|   TEXAS INSTRUMENTS INCORPORATED
|   Standard Linear and Logic
|   IBIS Model of SN74ALVC16835
|   18-BIT Universal Bus Driver with 3-state outputs
|   56-pin DGG, DGV, or DL Package
[IBIS Ver]   2.1
[Comment char]  |_char
[File Name]   alvc16835.ibs
[File Rev]   2.0
[Date]   6/17/97
[Source]   File originated at Texas Instruments, Inc.
[Notes]   The following is an IBIS list for the ALVC16835.
|   - This file may be incomplete or may not be fully compliant
|   with the IBIS specification. It will be replaced with a
|   version that is IBIS Revision 3.2 compliant and is complete
|   and accurate.  Please email all questions and comments to
|   sllibis@ti.com
|   - All test data contained in this file are derived from
|   hspice(tm) simulations.
|   - File created by Ramzi Ammar, SLL Applications
[Disclaimer]
* Property of Texas Instruments Incorporated.  Unauthorized *
* reproduction and/or distribution is strictly prohibited. *
* This product is protected under copyright law. *
* Created 1997, (C) Copyright 1997, Texas Instruments Inc., *
* All Rights Reserved *
* UNLESS THERE IS A SIGNED, WRITTEN AGREEMENT TO THE *
* CONTRARY, TEXAS INSTRUMENTS ("TI") IS PROVIDING THE IBIS *
* MODELS "AS IS" AND WITHOUT ANY WARRANTY, EXPRESSED OR *
* IMPLIED.  TI assumes no liability for: *
* 1) the accuracy of the IBIS models provided to your *
* company; *
* 2) the proper functioning of these IBIS models in your *
* design or for any resulting applications; or *
* 3) infringement of patents, copyrights or intellectual *
* property rights resulting from your use of these *
* IBIS models. *
* TI provides IBIS Models as a service to our customers. *
* You and your company shall not distribute, sell or give *
* these models to anyone else without prior written *
* permission from TI. *
* TI reserves the right to make changes to our products or *
* to discontinue any semiconductor product or service *
* without notice, and advises our customers to obtain the *
* latest version of relevant information to verify, before *
* placing orders, that the information being relied on is *
* current. *
* Please be aware that your receipt and use of the IBIS *
* information provided shall serve as acceptance of these *
* terms and conditions.  If you do not accept these terms, *
* you should return or destroy the IBIS models and any *
* other accompanying information immediately. *
[Component]   ALVC16835_DGG
[Manufacturer]  Texas Instruments, Inc.
[Package]
|   typ   min   max
R_pkg   0.045   0.035   0.062
L_pkg   3.324nH   2.403nH   5.094nH
C_pkg   0.564pF   0.341pF   0.914pF
[Pin]   signal_name   model_name   R_pin   L_pin   C_pin
1   NC   NC   0.062   5.094nH   0.856pF
2   NC   NC   0.061   4.621nH   0.902pF
3   Y1   OUT   0.06   4.316nH   0.802pF
4   GND   GND   0.059   3.968nH   0.698pF
5   Y2   OUT   0.057   3.716nH   0.649pF
6   Y3   OUT   0.042   3.517nH   0.652pF
7   VCC   POWER   0.041   3.16nH   0.57pF
8   Y4   OUT   0.039   2.981nH   0.482pF
9   Y5   OUT   0.039   2.809nH   0.447pF
10   Y6   OUT   0.038   2.715nH   0.409pF
11   GND   GND   0.041   2.675nH   0.391pF
12   Y7   OUT   0.039   2.536nH   0.366pF
13   Y8   OUT   0.039   2.457nH   0.348pF
14   Y9   OUT   0.038   2.411nH   0.353pF
15   Y10   OUT   0.039   2.456nH   0.355pF
16   Y11   OUT   0.039   2.471nH   0.349pF
17   Y12   OUT   0.04   2.58nH   0.37pF
18   GND   GND   0.038   2.651nH   0.389pF
19   Y13   OUT   0.038   2.739nH   0.411pF
20   Y14   OUT   0.039   2.838nH   0.449pF
21   Y15   OUT   0.038   2.988nH   0.484pF
22   VCC   POWER   0.038   3.105nH   0.564pF
23   Y16   OUT   0.04   3.427nH   0.638pF
24   Y17   OUT   0.056   3.654nH   0.641pF
25   GND   GND   0.057   3.932nH   0.7pF
26   Y18   OUT   0.058   4.257nH   0.806pF
27   OE_BAR   NC   0.057   4.58nH   0.914pF
28   LE   NC   0.059   5.038nH   0.861pF
29   GND   GND   0.06   5.058nH   0.858pF
30   CLK   NC   0.056   4.543nH   0.904pF
31   A18   IN   0.057   4.24nH   0.803pF
32   GND   GND   0.057   3.929nH   0.7pF
33   A17   IN   0.056   3.616nH   0.637pF
34   A16   IN   0.037   3.368nH   0.64pF
35   VCC   POWER   0.036   3.024nH   0.563pF
36   A15   IN   0.035   2.876nH   0.474pF
37   A14   IN   0.035   2.745nH   0.444pF
38   A13   IN   0.037   2.683nH   0.405pF
39   GND   GND   0.038   2.603nH   0.382pF
40   A12   IN   0.038   2.51nH   0.362pF
41   A11   IN   0.036   2.412nH   0.341pF
42   A10   IN   0.038   2.416nH   0.349pF
43   A9   IN   0.037   2.403nH   0.349pF
44   A8   IN   0.037   2.429nH   0.341pF
45   A7   IN   0.036   2.482nH   0.358pF
46   GND   GND   0.037   2.615nH   0.381pF
47   A6   IN   0.035   2.669nH   0.402pF
48   A5   IN   0.036   2.763nH   0.442pF
49   A4   IN   0.036   2.942nH   0.478pF
50   VCC   POWER   0.035   3.053nH   0.564pF
51   A3   IN   0.036   3.409nH   0.641pF
52   A2   IN   0.058   3.698nH   0.641pF
53   GND   GND   0.059   3.975nH   0.697pF
54   A1   IN   0.061   4.327nH   0.802pF
55   NC   NC   0.061   4.624nH   0.905pF
56   GND   GND   0.06   5.063nH   0.858pF
[Component]   ALVC16835_DGV
[Manufacturer]  Texas Instruments, Inc.
[Package]
|   typ   min   max
R_pkg   0.056   0.025   0.1
L_pkg   2.961nH   1.897nH   4.848nH
C_pkg   0.397pF   0.244pF   0.659pF
[Pin]   signal_name   model_name   R_pin   L_pin   C_pin
1   NC   NC   0.1   4.848nH   0.659pF
2   NC   NC   0.096   4.436nH   0.65pF
3   Y1   OUT   0.095   4.138nH   0.568pF
4   GND   GND   0.098   3.897nH   0.495pF
5   Y2   OUT   0.082   3.448nH   0.443pF
6   Y3   OUT   0.068   3.096nH   0.392pF
7   VCC   POWER   0.056   2.728nH   0.384pF
8   Y4   OUT   0.027   2.483nH   0.36pF
9   Y5   OUT   0.027   2.397nH   0.309pF
10   Y6   OUT   0.028   2.304nH   0.302pF
11   GND   GND   0.029   2.179nH   0.28pF
12   Y7   OUT   0.03   2.045nH   0.268pF
13   Y8   OUT   0.032   2.003nH   0.259pF
14   Y9   OUT   0.033   1.951nH   0.249pF
15   Y10   OUT   0.033   1.963nH   0.25pF
16   Y11   OUT   0.032   2.008nH   0.259pF
17   Y12   OUT   0.03   2.034nH   0.267pF
18   GND   GND   0.03   2.141nH   0.276pF
19   Y13   OUT   0.029   2.33nH   0.302pF
20   Y14   OUT   0.028   2.402nH   0.308pF
21   Y15   OUT   0.027   2.459nH   0.354pF
22   VCC   POWER   0.054   2.694nH   0.377pF
23   Y16   OUT   0.064   2.958nH   0.381pF
24   Y17   OUT   0.08   3.384nH   0.438pF
25   GND   GND   0.096   3.829nH   0.488pF
26   Y18   OUT   0.097   4.096nH   0.562pF
27   OE_BAR   NC   0.093   4.354nH   0.643pF
28   LE   NC   0.096   4.753nH   0.641pF
29   GND   GND   0.094   4.721nH   0.64pF
30   CLK   NC   0.089   4.276nH   0.633pF
31   A18   IN   0.089   4.015nH   0.555pF
32   GND   GND   0.096   3.852nH   0.488pF
33   A17   IN   0.079   3.379nH   0.438pF
34   A16   IN   0.065   2.984nH   0.384pF
35   VCC   POWER   0.054   2.682nH   0.375pF
36   A15   IN   0.026   2.451nH   0.353pF
37   A14   IN   0.026   2.334nH   0.302pF
38   A13   IN   0.028   2.289nH   0.297pF
39   GND   GND   0.027   2.104nH   0.272pF
40   A12   IN   0.029   2.009nH   0.263pF
41   A11   IN   0.031   1.955nH   0.254pF
42   A10   IN   0.031   1.902nH   0.245pF
43   A9   IN   0.031   1.897nH   0.244pF
44   A8   IN   0.03   1.955nH   0.254pF
45   A7   IN   0.029   2.024nH   0.265pF
46   GND   GND   0.028   2.133nH   0.275pF
47   A6   IN   0.028   2.305nH   0.299pF
48   A5   IN   0.027   2.376nH   0.305pF
49   A4   IN   0.025   2.47nH   0.359pF
50   VCC   POWER   0.056   2.72nH   0.383pF
51   A3   IN   0.064   2.983nH   0.387pF
52   A2   IN   0.081   3.408nH   0.441pF
53   GND   GND   0.095   3.872nH   0.492pF
54   A1   IN   0.098   4.142nH   0.564pF
55   NC   NC   0.096   4.428nH   0.64pF
56   GND   GND   0.095   4.772nH   0.649pF
[Component]   ALVC16835_DL
[Manufacturer]  Texas Instruments, Inc.
[Package]
|   typ   min   max
R_pkg   0.055   0.048   0.067
L_pkg   6.539nH   4.802nH   9.746nH
C_pkg   0.857pF   0.5pF   1.351pF
[Pin]   signal_name   model_name   R_pin   L_pin   C_pin
1   NC   NC   0.064   9.646nH   1.202pF
2   NC   NC   0.059   8.723nH   1.348pF
3   Y1   OUT   0.059   8.139nH   1.223pF
4   GND   GND   0.056   7.554nH   1.088pF
5   Y2   OUT   0.054   6.991nH   0.966pF
6   Y3   OUT   0.053   6.659nH   0.973pF
7   VCC   POWER   0.055   6.321nH   0.905pF
8   Y4   OUT   0.055   5.942nH   0.713pF
9   Y5   OUT   0.057   5.767nH   0.678pF
10   Y6   OUT   0.054   5.459nH   0.631pF
11   GND   GND   0.051   5.224nH   0.638pF
12   Y7   OUT   0.048   5.088nH   0.601pF
13   Y8   OUT   0.05   5.021nH   0.518pF
14   Y9   OUT   0.051   4.802nH   0.5pF
15   Y10   OUT   0.051   4.803nH   0.5pF
16   Y11   OUT   0.05   5.021nH   0.518pF
17   Y12   OUT   0.048   5.088nH   0.601pF
18   GND   GND   0.051   5.224nH   0.638pF
19   Y13   OUT   0.054   5.459nH   0.631pF
20   Y14   OUT   0.057   5.768nH   0.677pF
21   Y15   OUT   0.055   5.942nH   0.715pF
22   VCC   POWER   0.055   6.321nH   0.907pF
23   Y16   OUT   0.053   6.659nH   0.972pF
24   Y17   OUT   0.054   6.991nH   0.966pF
25   GND   GND   0.056   7.554nH   1.087pF
26   Y18   OUT   0.059   8.139nH   1.223pF
27   OE_BAR   NC   0.059   8.727nH   1.351pF
28   LE   NC   0.067   9.746nH   1.21pF
29   GND   GND   0.063   9.63nH   1.203pF
30   CLK   NC   0.06   8.751nH   1.349pF
31   A18   IN   0.06   8.184nH   1.224pF
32   GND   GND   0.056   7.543nH   1.087pF
33   A17   IN   0.054   7.005nH   0.969pF
34   A16   IN   0.056   6.714nH   0.975pF
35   VCC   POWER   0.058   6.384nH   0.909pF
36   A15   IN   0.057   5.976nH   0.717pF
37   A14   IN   0.057   5.743nH   0.677pF
38   A13   IN   0.055   5.469nH   0.631pF
39   GND   GND   0.055   5.328nH   0.644pF
40   A12   IN   0.052   5.189nH   0.606pF
41   A11   IN   0.052   5.053nH   0.519pF
42   A10   IN   0.052   4.825nH   0.502pF
43   A9   IN   0.054   4.896nH   0.506pF
44   A8   IN   0.052   5.093nH   0.521pF
45   A7   IN   0.051   5.179nH   0.608pF
46   GND   GND   0.054   5.314nH   0.645pF
47   A6   IN   0.055   5.511nH   0.632pF
48   A5   IN   0.057   5.77nH   0.677pF
49   A4   IN   0.055   5.956nH   0.716pF
50   VCC   POWER   0.055   6.32nH   0.905pF
51   A3   IN   0.052   6.621nH   0.968pF
52   A2   IN   0.053   6.974nH   0.966pF
53   GND   GND   0.057   7.571nH   1.089pF
54   A1   IN   0.057   8.097nH   1.219pF
55   NC   NC   0.059   8.723nH   1.349pF
56   GND   GND   0.061   9.56nH   1.199pF
| Models and submodels in the file (2): OUT (3-state), IN (Input)
